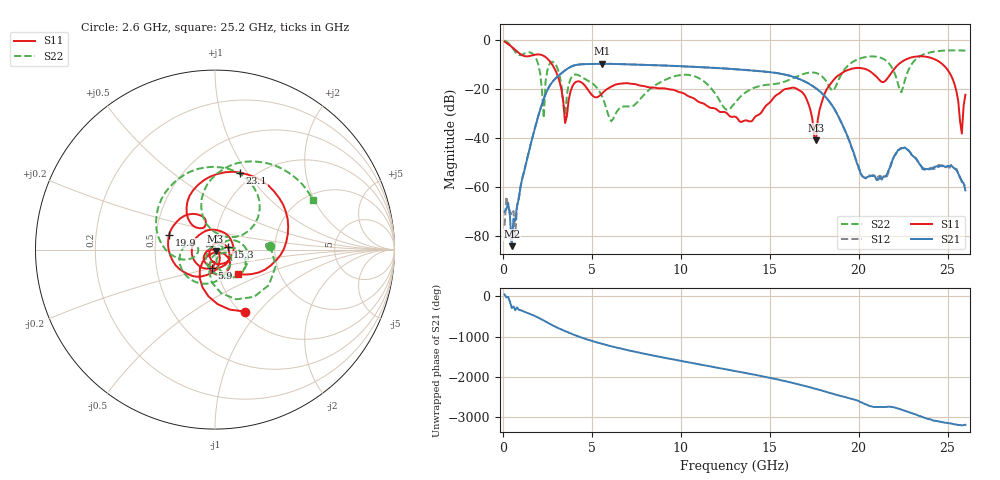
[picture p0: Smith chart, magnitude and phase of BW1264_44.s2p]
!Keysight Technologies,N5245B,MY57181159,A.13.60.06
!Date: Friday, December 18, 2020 23:54:23
!Correction: S11(Full 2 Port(1,2))
!S21(Full 2 Port(1,2))
!S12(Full 2 Port(1,2))
!S22(Full 2 Port(1,2))
!S2P File: Measurements: S11, S21, S12, S22:
# Hz S  dB  R 50
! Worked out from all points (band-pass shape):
!   260 points, 100 MHz to 26 GHz, reference 50 ohm
!   highest |S21| = -9.74 dB at 5.6 GHz (marker M1); lowest = -84.1 dB at 500 MHz (marker M2)
!   |S21| within 3 dB of the highest: 3.441 GHz to 14.45 GHz (11.01 GHz wide, 123 % of centre)
!   lowest |S11| = -41.0 dB at 17.6 GHz (marker M3), VSWR 1.02, Z = 50.3 - j0.848 ohm
!   |S11| at or under -10 dB: 2.769 GHz to 22.23 GHz (19.47 GHz wide, 156 % of centre); 24.72 GHz to end of sweep
!   |S22| runs from -33.2 to -0.2 dB; largest |S21 - S12| = 0.00054
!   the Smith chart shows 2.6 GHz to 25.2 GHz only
!   S11 on the Smith chart (normalised r, x): 2.6 GHz: 1.05, -0.84; 5.9 GHz: 0.95, -0.19; 15.3 GHz: 1.15, +0.03; 19.9 GHz: 0.59, +0.10; 23.1 GHz: 0.86, +0.93; 25.2 GHz: 1.24, -0.35
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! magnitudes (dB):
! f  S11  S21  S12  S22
! 100 MHz  -0.7  -70.1  -75.8  -0.2
! 500 MHz  -2.8  -84.1  -71.5  -2.9
! 700 MHz  -4.0  -73.7  -79.7  -4.9
! 1.9 GHz  -5.9  -33.4  -33.4  -8.1
! 2.3 GHz  -6.5  -24.0  -24.1  -31.9
! 2.6 GHz  -8.4  -19.1  -19.1  -10.2
! 3.5 GHz  -33.9  -12.4  -12.4  -32.6
! 4.5 GHz  -17.8  -9.9  -9.9  -15.4
! 5.6 GHz  -21.7  -9.7  -9.7  -23.4
! 5.9 GHz  -19.8  -9.7  -9.7  -30.0
! 8.8 GHz  -19.7  -10.4  -10.4  -17.5
! 13.1 GHz  -31.4  -12.0  -12.0  -25.2
! 15.3 GHz  -23.0  -13.4  -13.4  -18.0
! 17.4 GHz  -32.4  -18.7  -18.7  -13.3
! 17.6 GHz  -41.0  -19.7  -19.7  -13.5
! 18.2 GHz  -20.2  -23.8  -23.8  -17.1
! 19.9 GHz  -11.4  -50.2  -49.8  -8.0
! 21.7 GHz  -14.9  -52.9  -53.6  -9.5
! 23.1 GHz  -6.9  -47.7  -47.7  -8.7
! 25.2 GHz  -14.6  -51.1  -51.3  -4.3
! 25.8 GHz  -38.2  -58.0  -57.4  -4.3
! 26 GHz  -22.4  -61.4  -59.5  -4.3
